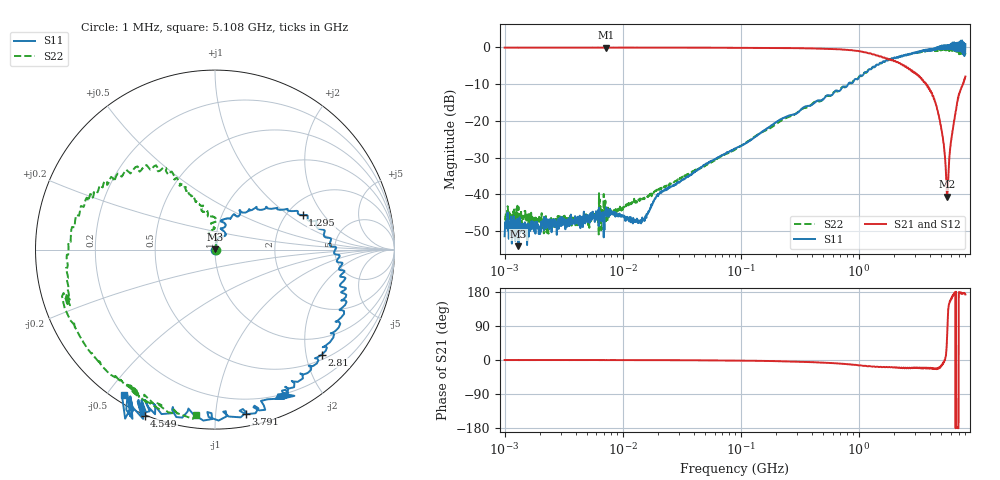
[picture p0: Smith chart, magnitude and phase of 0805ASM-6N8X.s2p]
!s-Parameter Generated by FASTRON Sdn. Bhd.
!FASTRON P/N : 0805ASM-6N8X
!Keysight Technologies: E5071C_MY46733604_B.14.02
!Date: Fri Jun 19 14:46:49 2026
!Version  :Rev00  Fri Jun 19 14:46:49 2026
!Data & Calibration Information:
!Freq  S11:SOLT2(ON)  S21:SOLT2(ON)  S12:SOLT2(ON)  S22:SOLT2(ON)
!PortZ  Port1:50+j0  Port2:50+j0
!When reading reference impedance value at option line is always used.
! Remarks : This data is being provided solely for informational purposes.
# Hz S dB R 50
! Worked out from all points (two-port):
!   1601 points, 1 MHz to 8 GHz, reference 50 ohm
!   highest |S21| = -0.02 dB at 7.229 MHz (marker M1); lowest = -40.6 dB at 5.612 GHz (marker M2)
!   |S21| within 3 dB of the highest: start of sweep to 1.696 GHz; 1.704 GHz to 1.754 GHz (49.4 MHz wide, 2.86 % of centre)
!   lowest |S11| = -54.1 dB at 1.31 MHz (marker M3), VSWR 1.00, Z = 50 + j0.195 ohm
!   |S11| at or under -10 dB: start of sweep to 813.3 MHz
!   |S22| runs from -50.9 to -0.4 dB; largest |S21 - S12| = 0.011
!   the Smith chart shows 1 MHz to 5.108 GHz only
!   S11 on the Smith chart (normalised r, x): 1 MHz: 1.01, -0.00; 1.295 GHz: 2.42, +1.28; 2.81 GHz: 0.60, -2.31; 3.791 GHz: 0.08, -1.20; 4.549 GHz: -0.00, -0.66; 5.108 GHz: 0.03, -0.55
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1000000  -51.40 -18.8  -0.05 -0.1  -0.04 -0.1  -47.00 -1.4
1310238  -54.10 98.7  -0.09 0.1  -0.06 -0.1  -43.40 -21.8
2248791  -48.70 9.6  -0.04 -0.1  -0.05 -0.1  -48.20 10.2
4479405  -47.40 18.0  -0.05 -0.1  -0.05 -0.2  -47.50 26.9
7228921  -43.50 39.2  -0.02 -0.2  -0.06 -0.1  -47.30 58.6
1.414737e7  -47.00 56.7  -0.04 -0.3  -0.06 -0.3  -41.30 46.9
2.00676e7  -39.90 59.0  -0.05 -0.4  -0.06 -0.3  -38.80 65.1
8.994653e7  -27.50 77.5  -0.07 -1.5  -0.09 -1.5  -27.70 80.0
4.006501e8  -15.60 77.9  -0.26 -5.6  -0.26 -5.6  -15.40 87.8
7.847468e8  -10.70 48.7  -0.62 -10.9  -0.62 -11.0  -10.50 112.0
1.295411e9  -5.61 21.5  -1.85 -17.4  -1.84 -17.5  -5.49 121.0
1.7949e9  -3.26 -2.4  -3.28 -18.6  -3.28 -18.9  -3.25 142.0
2.384191e9  -2.15 -21.3  -4.90 -20.2  -4.98 -20.5  -2.24 159.0
2.809687e9  -1.57 -44.5  -6.21 -21.0  -6.29 -21.0  -1.76 -179.0
3.791269e9  -0.60 -79.5  -10.30 -22.0  -10.20 -22.2  -0.96 -147.0
4.548578e9  0.04 -113.0  -15.90 -22.6  -15.90 -22.9  -0.93 -122.0
5.108415e9  -0.37 -122.0  -24.00 -10.8  -24.00 -11.1  -0.63 -96.7
5.612268e9  0.18 -144.0  -40.60 77.4  -40.60 77.1  -0.87 -64.2
6.110812e9  0.83 -145.0  -24.50 165.0  -24.60 164.0  -0.77 -54.5
6.65058e9  -0.09 -156.0  -17.20 180.0  -17.10 179.0  -0.62 -3.3
7.306013e9  1.85 179.0  -11.40 177.0  -11.20 177.0  -1.09 6.7
8e9  0.87 148.0  -7.91 173.0  -7.79 173.0  -1.51 42.2
